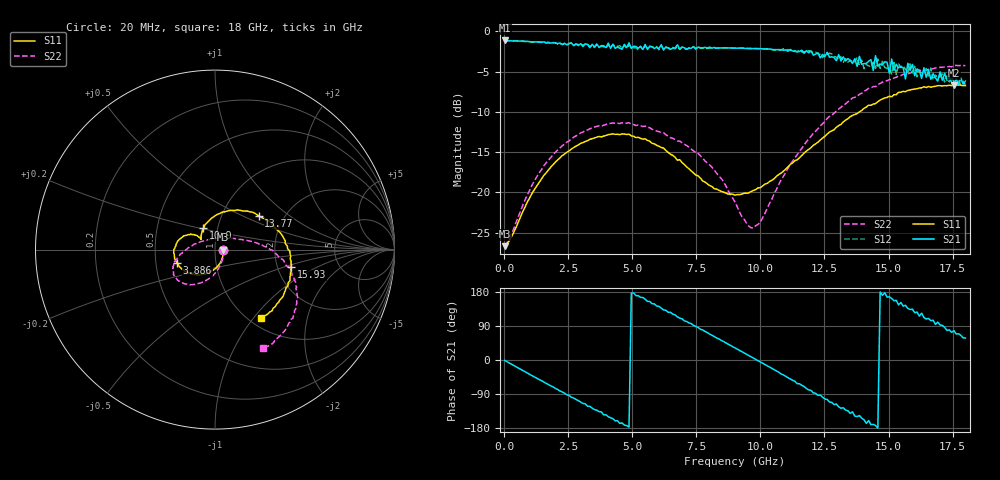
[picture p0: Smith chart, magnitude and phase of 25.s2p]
!Agilent Technologies,N5230A,US43500223,A.07.50.48
!Agilent N5230A: A.07.50.48
!Date: Saturday, January 16, 2016 18:00:10
!Correction: S11(Full 2 Port(1,2))
!S21(Full 2 Port(1,2))
!S12(Full 2 Port(1,2))
!S22(Full 2 Port(1,2))
!S2P File: Measurements: S11, S21, S12, S22:
# Hz S  dB  R 50
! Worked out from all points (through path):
!   201 points, 20 MHz to 18 GHz, reference 50 ohm
!   highest |S21| = -1.14 dB at 20 MHz (marker M1); lowest = -6.7 dB at 17.55 GHz (marker M2)
!   group delay of S21, straight-line fit = 103 ps
!   lowest |S11| = -26.7 dB at 20 MHz (marker M3), VSWR 1.10, Z = 54.8 - j0.122 ohm
!   |S11| at or under -10 dB: start of sweep to 13.87 GHz
!   |S22| runs from -26.7 to -4.2 dB; largest |S21 - S12| = 0.14
!   S11 on the Smith chart (normalised r, x): 20 MHz: 1.10, -0.00; 3.886 GHz: 0.65, -0.10; 10.9 GHz: 0.86, +0.21; 13.77 GHz: 1.49, +0.62; 15.93 GHz: 2.37, -0.58; 18 GHz: 1.14, -1.10
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2e7  -26.70 -1.4  -1.14 -0.8  -1.15 -0.9  -26.65 -2.5
1.5483e9  -17.91 -101.9  -1.31 -58.0  -1.30 -58.2  -16.70 -94.8
3.0766e9  -13.83 -142.7  -1.89 -114.7  -1.80 -114.2  -12.51 -124.4
3.8857e9  -13.02 -160.5  -1.80 -144.7  -1.90 -143.9  -11.67 -136.5
4.8746e9  -12.79 179.7  -1.44 -176.9  -1.67 -177.1  -11.35 -149.3
6.0433e9  -14.29 157.8  -2.15 141.5  -2.30 141.0  -12.47 -162.4
6.7625e9  -16.02 147.6  -1.67 113.8  -1.90 113.6  -13.63 -169.0
7.5716e9  -17.97 141.8  -1.96 86.0  -1.91 85.5  -15.16 -177.5
9.01e9  -20.35 143.5  -2.08 31.9  -2.10 31.8  -21.20 148.3
9.7292e9  -19.77 139.4  -2.15 5.0  -2.15 4.8  -24.43 94.4
1.08979e10  -17.38 118.5  -2.36 -39.2  -2.17 -39.8  -18.03 29.1
1.20666e10  -14.16 86.8  -2.97 -86.7  -2.65 -84.4  -12.68 9.5
1.2606e10  -12.77 70.6  -2.61 -104.0  -2.99 -106.1  -10.83 2.8
1.37747e10  -10.23 37.6  -4.35 -149.2  -3.24 -151.2  -8.10 -10.4
1.4404e10  -9.04 21.1  -4.87 -169.9  -3.83 -171.0  -6.86 -18.3
1.44939e10  -8.99 19.6  -3.03 -172.9  -4.61 -171.5  -6.88 -18.7
1.50333e10  -8.07 6.7  -5.20 166.9  -4.58 162.3  -5.99 -24.9
1.51232e10  -8.14 5.3  -3.45 162.3  -5.33 166.1  -6.03 -25.5
1.59323e10  -7.22 -13.1  -4.12 134.2  -5.15 130.6  -5.09 -35.6
1.66515e10  -6.95 -28.2  -5.96 103.9  -4.57 104.7  -4.72 -45.0
1.75505e10  -6.63 -46.9  -6.73 77.6  -6.22 69.9  -4.29 -57.5
1.8e10  -6.75 -55.8  -6.20 57.9  -6.65 56.8  -4.25 -63.9
